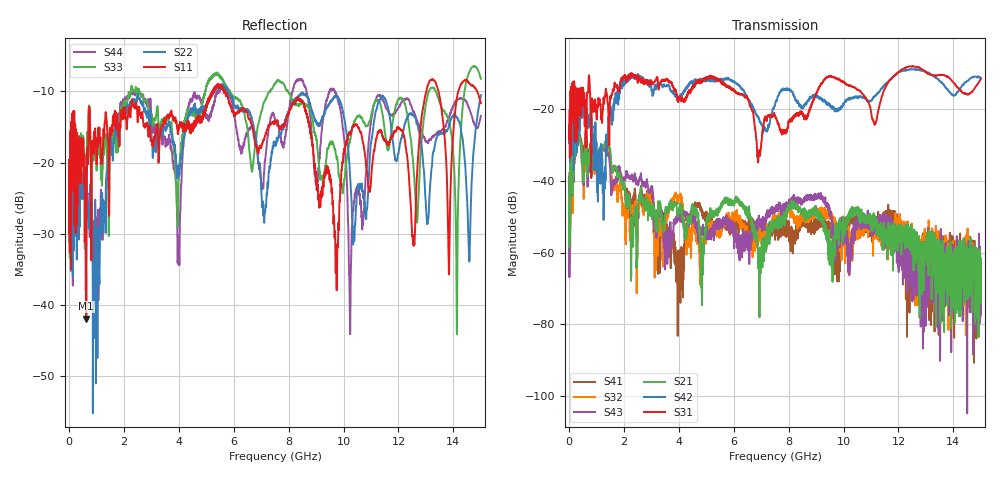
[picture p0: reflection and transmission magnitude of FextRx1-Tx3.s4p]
! FILE: N:\QM 2007\Prüfprotokolle\Highspeed\Konfektionierte Ltg\L45593-D106\D30\8216\0002\Fext\FextRx1-Tx3.s4p
# MHz S DB R 50.00
! FREQ  S11  S12  S13  S14
!  S21  S22  S23  S24
!  S31  S32  S33  S34
!  S41  S42  S43  S44
!  DB  ANG  DB  ANG  DB  ANG  DB  ANG
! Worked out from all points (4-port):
!   2999 points, 10 MHz to 15 GHz, reference 50 ohm
!   strongest paths, dB at 10 MHz, 3.755 GHz, 7.505 GHz, 11.26 GHz, 15 GHz:
!     S31: -25.5, -12.8, -21.9, -20.7, -11.5
!     S42: -24.4, -15.2, -18.8, -15.6, -11.4
!     S21: -43.5, -47.5, -52.5, -54.7, -68.4
!     S43: -43.4, -57.0, -48.7, -52.1, -66.3
!     S32: -48.2, -45.3, -51.0, -54.8, -69.4
!     S41: -43.9, -56.1, -56.4, -52.9, -67.2
!   lowest |S11| = -41.9 dB at 635 MHz (marker M1), VSWR 1.02, Z = 50.4 + j0.683 ohm
!   |S11| at or under -10 dB: start of sweep to 5.223 GHz; 5.697 GHz to 13.01 GHz (7.318 GHz wide, 78.2 % of centre); 13.46 GHz to 14.18 GHz (722.1 MHz wide, 5.23 % of centre)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
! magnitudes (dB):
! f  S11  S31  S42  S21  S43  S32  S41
! 10 MHz  -19.6  -25.5  -24.4  -43.5  -43.4  -48.2  -43.9
! 635 MHz  -41.9  -29.9  -21.7  -28.5  -27.5  -28.6  -26.4
! 4.025 GHz  -14.6  -17.0  -17.0  -47.4  -49.9  -44.1  -65.7
! 9.735 GHz  -34.7  -11.5  -20.1  -53.3  -57.0  -54.1  -58.6
! 10.24 GHz  -15.9  -13.5  -16.9  -48.4  -62.7  -54.3  -51.3
! 14.12 GHz  -11.1  -13.7  -15.4  -73.3  -58.7  -66.8  -60.7
! 15 GHz  -11.6  -11.5  -11.4  -68.4  -66.3  -69.4  -67.2
